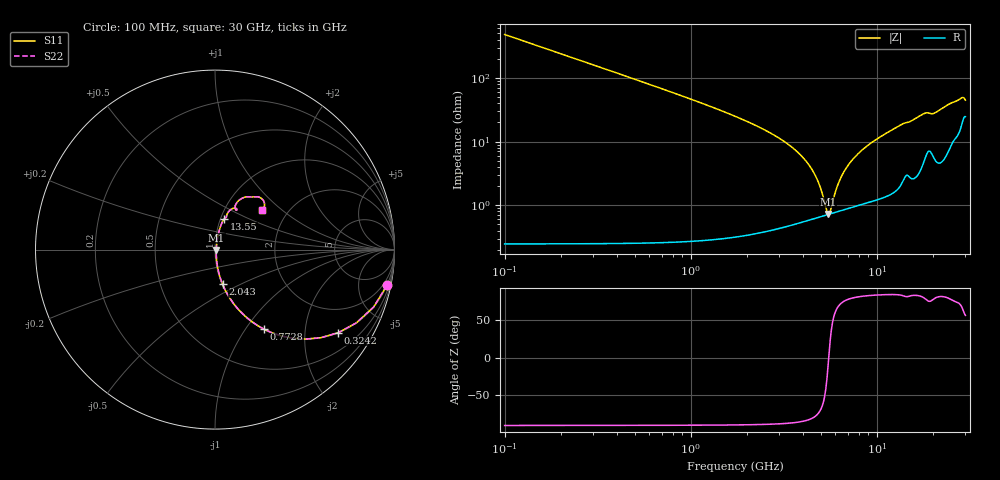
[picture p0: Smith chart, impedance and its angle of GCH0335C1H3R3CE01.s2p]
!Murata Part Number: GCH0335C1H3R3CE01
!These Parameters are Measured in Series Mode Connection
!Data Generated on Jun 19, 2026
!  o--ll--o
!Port1  Port2
!  o------o
!Operation Temp=25[degC], DC Bias Voltage=0[V]
!Freq. Start=100[MHz] Stop=30[GHz] 401[Steps]
# Hz S RI R 50
!Freq.(Hz) S11(Real) S11(Imag) S21(Real) S21(Imag) S12(Real) S12(Imag) S22(Real) S22(Imag)
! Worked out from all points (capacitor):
!   401 points, 100 MHz to 30 GHz, reference 50 ohm
!   read as one part in series: C = 3.3 pF near 249.5 MHz
!   lowest |Z| = 729 mohm at 5.482 GHz (marker M1)
!   series resonance near 5.525 GHz, so ESL is about 250 pH
!   S11 on the Smith chart (normalised r, x): 100 MHz: 1.00, -9.64; 324.2 MHz: 1.00, -2.96; 772.8 MHz: 1.01, -1.22; 2.043 GHz: 1.01, -0.41; 13.55 GHz: 1.04, +0.37; 30 GHz: 1.49, +0.75
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1e8  0.9587 -0.1988  0.0413 0.1988  0.0413 0.1988  0.9587 -0.1988
3.2425e8  0.6869 -0.4629  0.3131 0.4629  0.3131 0.4629  0.6869 -0.4629
4.7375e8  0.5051 -0.4987  0.4949 0.4987  0.4949 0.4987  0.5051 -0.4987
7.7275e8  0.2731 -0.4434  0.7269 0.4434  0.7269 0.4434  0.2731 -0.4434
1.22125e9  0.1252 -0.3272  0.8748 0.3272  0.8748 0.3272  0.1252 -0.3272
2.0435e9  0.0425 -0.1936  0.9575 0.1936  0.9575 0.1936  0.0425 -0.1936
4.1365e9  0.00808 -0.0499  0.9919 0.0499  0.9919 0.0499  0.00808 -0.0499
4.65975e9  0.00702 -0.0291  0.993 0.0291  0.993 0.0291  0.00702 -0.0291
5.10825e9  0.00686 -0.0133  0.9931 0.0133  0.9931 0.0133  0.00686 -0.0133
5.482e9  0.00711 -0.00133  0.9929 0.00133  0.9929 0.00133  0.00711 -0.00133
5.6315e9  0.00729 0.00323  0.9927 -0.00323  0.9927 -0.00323  0.00729 0.00323
6.30425e9  0.00853 0.0223  0.9915 -0.0223  0.9915 -0.0223  0.00853 0.0223
7.05175e9  0.0106 0.0414  0.9894 -0.0414  0.9894 -0.0414  0.0106 0.0414
8.3225e9  0.0152 0.0704  0.9848 -0.0704  0.9848 -0.0704  0.0152 0.0704
1.01165e10  0.0238 0.1069  0.9762 -0.1069  0.9762 -0.1069  0.0238 0.1069
1.3555e10  0.0514 0.1704  0.9486 -0.1704  0.9486 -0.1704  0.0514 0.1704
1.505e10  0.0635 0.1855  0.9365 -0.1855  0.9365 -0.1855  0.0635 0.1855
1.796525e10  0.1061 0.2311  0.8939 -0.2311  0.8939 -0.2311  0.1061 0.2311
2.005825e10  0.1129 0.2251  0.8871 -0.2251  0.8871 -0.2251  0.1129 0.2251
2.50665e10  0.1851 0.2946  0.8149 -0.2946  0.8149 -0.2946  0.1851 0.2946
2.86545e10  0.2629 0.2815  0.7371 -0.2815  0.7371 -0.2815  0.2629 0.2815
3e10  0.2639 0.2209  0.7361 -0.2209  0.7361 -0.2209  0.2639 0.2209
